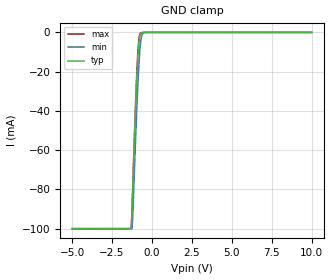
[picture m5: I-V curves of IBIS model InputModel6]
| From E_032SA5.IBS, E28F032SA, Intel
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|*************************Input Model 6****************************
[Model]   InputModel6
Model_type   Input
|   For CE#6
Vinl = 0.8V
Vinh = 2.0V
| Variable   typ   min   max
C_comp   5.61p   NA   7.6p
[Voltage Range]   5.0V   4.5V   5.5V
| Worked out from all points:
|   GND clamp passes 1 mA (typ) near -0.73 V on its own axis
[GND_clamp]
|Voltage I(typ)   I(min)   I(max)
-5V       -100mA     -100mA     -100mA
-1.3V     -100mA     -100mA     -100mA
-1.25V    -92.01mA   -100mA     -89.31mA
-1.2V     -79.25mA   -93.18mA   -76.71mA
-1.05V    -43.73mA   -59.3mA    -40.58mA
-950mV    -22.93mA   -38.64mA   -20.01mA
-900mV    -14.44mA   -29.19mA   -11.69mA
-800mV    -3.479mA   -13.68mA   -2.136mA
-700mV    -424.7uA   -4.142mA   -264uA
-600mV    -81.44uA   -742.3uA   -70.86uA
-500mV    -13.16uA   -96.1uA    -10.17uA
10V       0A         0A         0A
[POWER_clamp]
| Input buffer circuits of this product do not intrinsically
| require a [POWER_clamp] definition.  This zero current
| [POWER_clamp] is provided for compatibility with some ibis
| parsers.
|   Voltage  I(typ)   I(min)   I(max)
-5V       0A         0A         0A
-4.75V    0A         0A         0A
9.75V     0A         0A         0A
10V       0A         0A         0A
